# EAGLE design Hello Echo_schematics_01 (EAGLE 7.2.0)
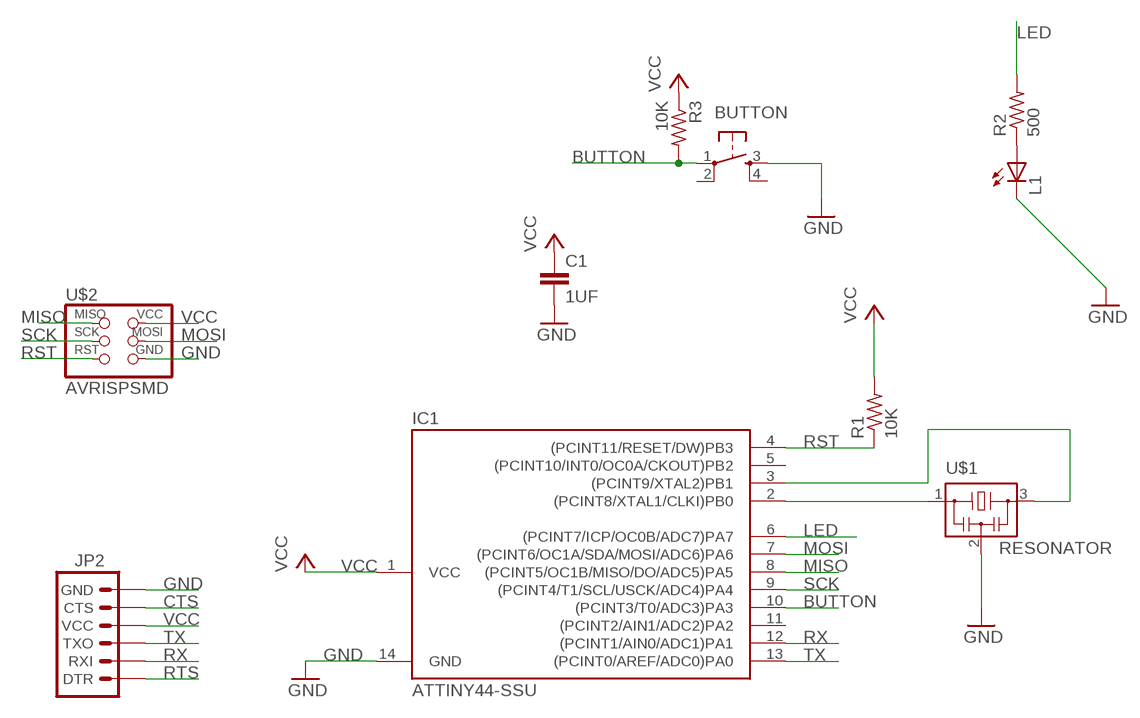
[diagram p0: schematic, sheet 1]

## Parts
BUTTON  6MM_SWITCH6MM_SWITCH  [6MM_SWITCH]
C1  1UF  CAP1206  [1206]
IC1  ATTINY44-SSU  [SOIC14]
JP2  ARDUINO_SERIAL_PROGRAMSMD  [1X06-SMD]
L1  LED1206  [1206]
R1  10K  RESISTOR1206  [1206]
R2  500  RESISTOR1206  [1206]
R3  10K  RESISTOR1206  [1206]
U$1  RESONATOR  [EFOBM]
U$2  AVRISPSMD  [2X03SMD]

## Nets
BUTTON: BUTTON.1(P) IC1.10((PCINT3/T0/ADC3)PA3) R3.2
CTS: JP2.5(CTS)
GND: BUTTON.3(S) C1.2 IC1.14(GND) JP2.6(GND) L1.2(C) U$1.2 U$2.6(GND)
LED: IC1.6((PCINT7/ICP/OC0B/ADC7)PA7) R2.2
MISO: IC1.8((PCINT5/OC1B/MISO/DO/ADC5)PA5) U$2.1(MISO)
MOSI: IC1.7((PCINT6/OC1A/SDA/MOSI/ADC6)PA6) U$2.4(MOSI)
N$1: IC1.2((PCINT8/XTAL1/CLKI)PB0) U$1.1
N$2: L1.1(A) R2.1
N$3: IC1.3((PCINT9/XTAL2)PB1) U$1.3
RST: IC1.4((PCINT11/RESET/DW)PB3) R1.1 U$2.5(RST)
RTS: JP2.1(DTR)
RX: IC1.12((PCINT1/AIN0/ADC1)PA1) JP2.2(RXI)
SCK: IC1.9((PCINT4/T1/SCL/USCK/ADC4)PA4) U$2.3(SCK)
TX: IC1.13((PCINT0/AREF/ADC0)PA0) JP2.3(TXO)
VCC: C1.1 IC1.1(VCC) JP2.4(VCC) R1.2 R3.1 U$2.2(VCC)
Unconnected: BUTTON.2(P1) BUTTON.4(S1) IC1.5((PCINT10/INT0/OC0A/CKOUT)PB2) IC1.11((PCINT2/AIN1/ADC2)PA2)

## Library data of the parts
BUTTON = 01_FAB_Hello:6MM_SWITCH: OMRON SWITCH
C1 = 01_SparkFun:CAP: Capacitor
IC1 = 01_FAB_Hello:ATTINY44
JP2 = 01_SparkFun:ARDUINO_SERIAL_PROGRAM
L1 = 01_FAB_Hello:LED
R1-R3 = 01_FAB_Hello:RESISTOR
U$1 = 01_fab:RESONATOR
U$2 = 01_FAB_Hello:AVRISP

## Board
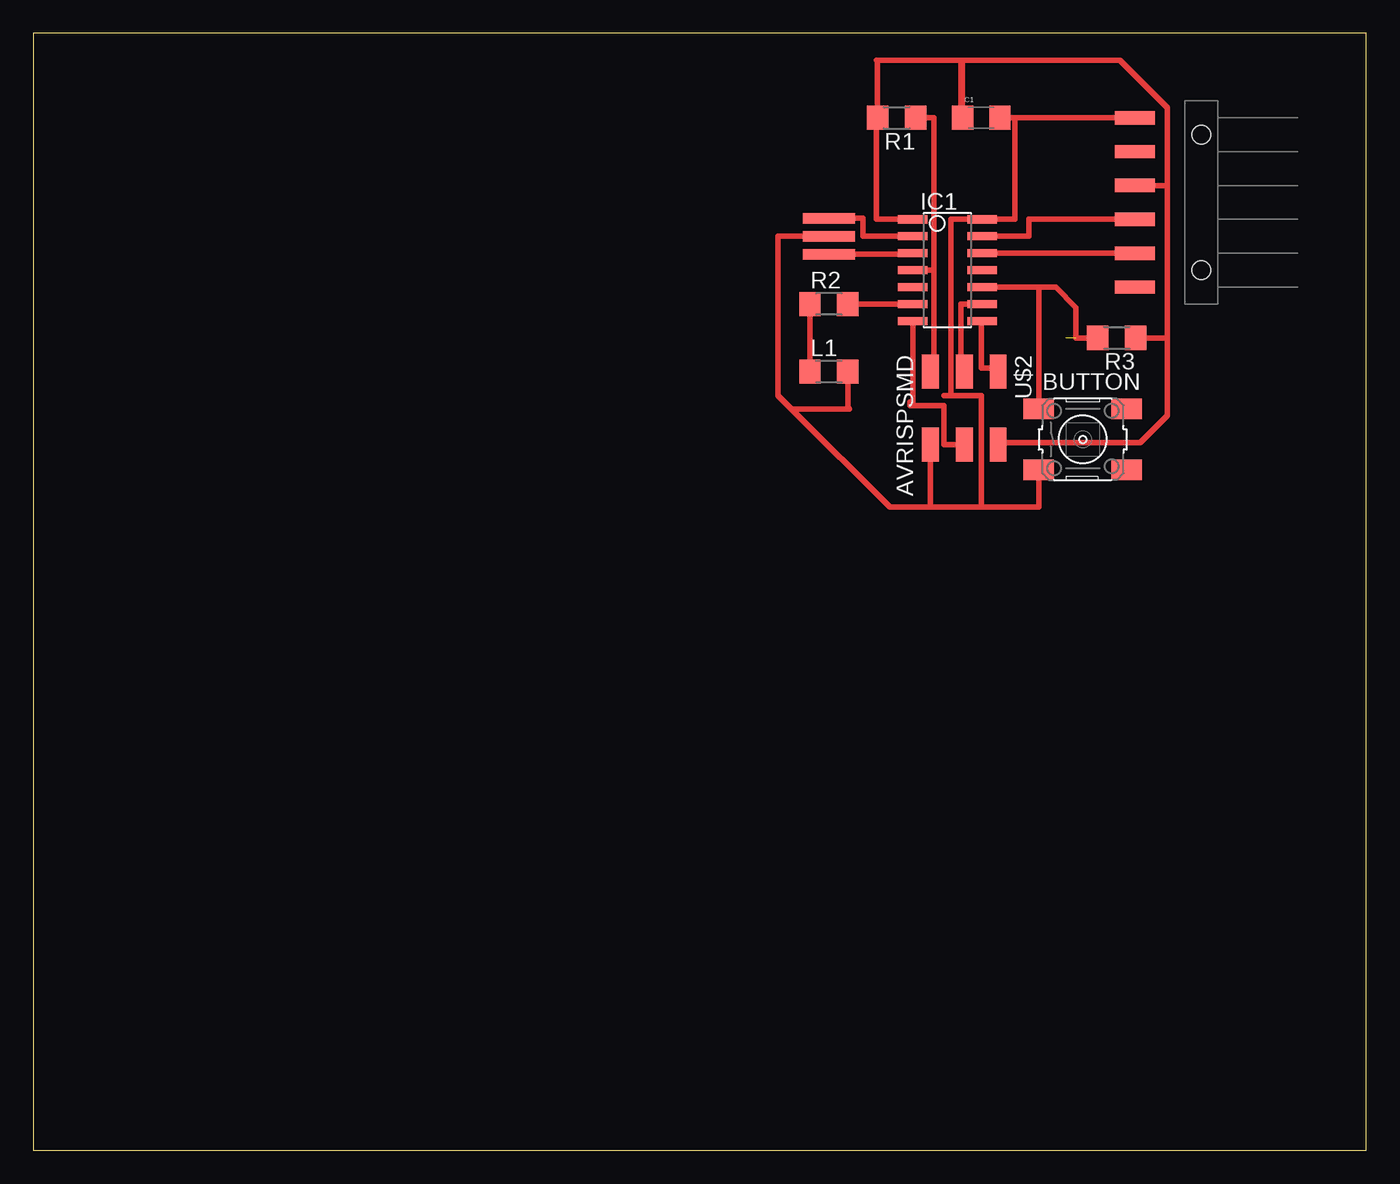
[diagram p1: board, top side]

Size 100 x 83.81 mm. Coordinates in mm from the lower left corner, seen from the top.
Outline: 0,0 100,0 100,83.81 0,83.81 0,0
Copper layers (1*16): Top 0.035mm / dielectric 1.5mm / Bottom 0.035mm
Design rules "default": minimum track width 10mil, minimum drill 24mil, track to track 8mil, track to pad 8mil, pad to pad 8mil, via to via 8mil, smd to smd 8mil, copper to edge 40mil, drill to drill 8mil, minimum pad ring 10mil, minimum via ring 8mil, stop-mask expansion 4mil, vias tented up to drill 0mil, thermal gap 10mil

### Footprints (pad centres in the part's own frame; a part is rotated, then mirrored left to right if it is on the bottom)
6MM_SWITCH = smd 2.286 x 1.524: 1 -3.302,2.286; 2 3.302,2.286; 3 -3.302,-2.286; 4 3.302,-2.286
1206 = smd 1.6 x 1.8: 1 -1.4,0; 2 1.4,0
SOIC14 = smd 0.61 x 2.21: 1 -3.81,-2.603; 2 -2.54,-2.603; 3 -1.27,-2.603; 4 0,-2.603; 5 1.27,-2.603; 6 2.54,-2.603; 7 3.81,-2.603; 8 3.81,2.603; 9 2.54,2.603; 10 1.27,2.603; 11 0,2.603; 12 -1.27,2.603; 13 -2.54,2.603; 14 -3.81,2.603
1X06-SMD = smd 1 x 3: 1 -6.35,5; 2 -3.81,5; 3 -1.27,5; 4 1.27,5; 5 3.81,5; 6 6.35,5 | hole 1.4: -5.08,0; 5.08,0
1206' = smd 1.6 x 1.803: 1 -1.422,0; 2 1.422,0
EFOBM = smd 0.8 x 3.9: 1 -1.35,0; 2 0,0; 3 1.35,0
2X03SMD = smd 2.54 x 1.27: 1 -2.54,2.54; 2 2.92,2.54; 3 -2.54,0; 4 2.92,0; 5 -2.54,-2.54; 6 2.92,-2.54

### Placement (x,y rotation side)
BUTTON  78.74,53.34 0 top
C1  71.12,77.47 0 top
IC1  68.58,66.04 270 top
JP2  87.63,71.12 90 top
L1  [1206']  59.69,58.42 0 top
R1  10K  [1206']  64.77,77.47 180 top
R2  500  [1206']  59.69,63.5 0 top
R3  10K  [1206']  81.28,60.96 180 top
U$1  59.69,68.58 270 top
U$2  69.85,55.88 270 top

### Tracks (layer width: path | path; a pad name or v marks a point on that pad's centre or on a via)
BUTTON  (1 unrouted)
  Top 0.406: R3.2 78.23,60.96 78.23,63.25 76.71,64.77 IC1.10 75.44,64.77 BUTTON.1
GND
  Top 0.406: JP2.6 C1.2 73.66,77.47 73.66,69.85 IC1.14 68.83,69.85 68.83,56.64 | U$1.2 55.88,68.58 55.88,56.64 56.9,55.63 | 71.12,48.26 75.44,48.26 BUTTON.3 | 71.12,48.26 67.31,48.26 | 67.31,48.26 U$2.6 | 68.33,56.64 68.83,56.64 | 68.83,56.64 71.12,56.64 71.12,48.26 | 56.9,55.63 64.26,48.26 67.31,48.26 | 56.9,55.63 61.21,55.63 61.11,55.73 L1.2
LED
  Top 0.406: R2.2 IC1.6
MISO
  Top 0.406: IC1.8 71.12,62.23 71.12,58.67 72.39,58.67 U$2.1
MOSI
  Top 0.406: U$2.4 68.33,52.96 68.33,55.88 65.79,55.88 65.79,56.13 65.98,56.13 IC1.7
N$1
  Top 0.406: U$1.1 62.23,69.93 62.23,68.58 IC1.2
N$2
  Top 0.406: R2.1 L1.1
N$3
  Top 0.406: U$1.3 65.98,67.23 IC1.3
RST
  Top 0.406: R1.1 67.56,77.47 67.56,66.04 | IC1.4 67.56,66.04 | 67.56,66.04 67.56,58.93 67.31,58.93 U$2.5
RX
  Top 0.406: JP2.2 IC1.12
SCK
  Top 0.406: U$2.3 69.6,58.42 69.6,63.5 IC1.9
TX
  Top 0.406: JP2.3 74.68,69.85 74.68,68.58 IC1.13
VCC
  Top 0.406: C1.1 69.85,77.47 | 63.35,80.01 R1.2 | JP2.4 85.09,72.39 | 85.09,72.39 85.09,60.96 | 85.09,60.96 R3.1 | R1.2 63.25,77.47 63.25,69.85 IC1.1 | U$2.2 72.52,53.09 83.06,53.09 85.09,55.12 85.09,60.96 | 85.09,72.39 85.09,78.23 81.53,81.79 69.72,81.79 C1.1 | 63.25,81.79 63.35,81.69 | 63.35,81.69 R1.2 | C1.1 69.6,77.47 69.6,81.79 63.35,81.79 63.35,81.69

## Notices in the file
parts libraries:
01_SparkFun: Licensing: CC v3.0 Share-Alike You are welcome to use this library for commercial purposes.
